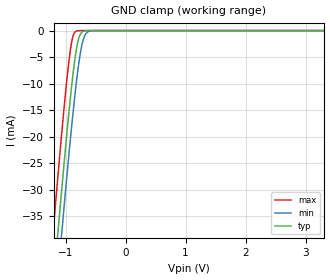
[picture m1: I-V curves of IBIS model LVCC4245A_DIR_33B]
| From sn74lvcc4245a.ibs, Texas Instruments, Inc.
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[Model]   LVCC4245A_DIR_33B
Model_type  Input
Vinl=0.8
Vinh=2.0
| variable   typ   min   max
C_comp   3.07pF   2.52pF   3.92pF
[Temperature Range]   40   100   -40
| Ambient temperature   25   85   -40
[Voltage range]   3.3   2.7   3.6
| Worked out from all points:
|   GND clamp passes 1 mA (typ) near -0.77 V on its own axis
[GND Clamp]
| LVCC4245A_DIR_33B
|   Voltage   I(typ)   I(min)   I(max)
-3.3V     -341.9mA   -349.3mA   -332.6mA
-1.215V   -49.65mA   -57.94mA   -39mA
-1.185V   -45.67mA   -53.97mA   -35.02mA
-1.125V   -37.81mA   -46.11mA   -27.16mA
-1.065V   -30.11mA   -38.37mA   -19.53mA
-920mV    -12.76mA   -20.55mA   -3.722mA
-875mV    -8.133mA   -15.46mA   -1.066mA
-825mV    -3.926mA   -10.27mA   -137.3uA
-775mV    -1.292mA   -5.836mA   -13.58uA
-715mV    -205.6uA   -2.13mA    -809.4nA
-585mV    -2.269uA   -70.9uA    -1.787nA
3.3V      4.879pA    7.789pA    4.387pA
